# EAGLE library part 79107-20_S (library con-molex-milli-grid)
RECEPTACAL
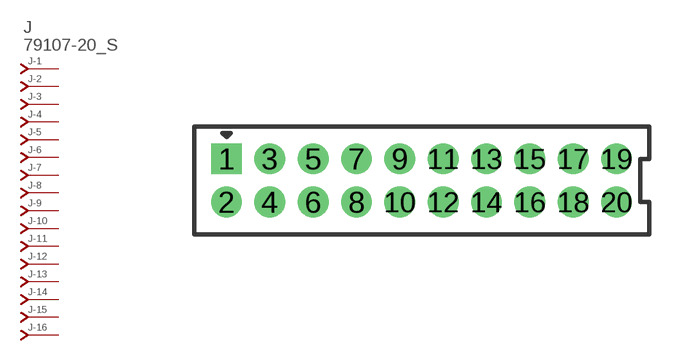
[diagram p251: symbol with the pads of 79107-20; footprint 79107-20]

Designator prefix J; gates -1=J-NV -2=J-N -3=J-N -4=J-N -5=J-N -6=J-N -7=J-N -8=J-N -9=J-N -10=J-N -11=J-N -12=J-N -13=J-N -14=J-N -15=J-N -16=J-N -17=J-N -18=J-N -19=J-N -20=J-N

## 79107-20_S  [79107-20]
1  -1:J  pas
2  -2:J  pas
3  -3:J  pas
4  -4:J  pas
5  -5:J  pas
6  -6:J  pas
7  -7:J  pas
8  -8:J  pas
9  -9:J  pas
10  -10:J  pas
11  -11:J  pas
12  -12:J  pas
13  -13:J  pas
14  -14:J  pas
15  -15:J  pas
16  -16:J  pas
17  -17:J  pas
18  -18:J  pas
19  -19:J  pas
20  -20:J  pas

## Footprint 79107-20 (pad centres in mm)
RECEPTACAL Dual Row, Vertical, Through-Hole
drill 0.914 square: 1 -9,1
drill 0.914: 2 -9,-1; 3 -7,1; 4 -7,-1; 5 -5,1; 6 -5,-1; 7 -3,1; 8 -3,-1; 9 -1,1; 10 -1,-1; 11 1,1; 12 1,-1; 13 3,1; 14 3,-1; 15 5,1; 16 5,-1; 17 7,1; 18 7,-1; 19 9,1; 20 9,-1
